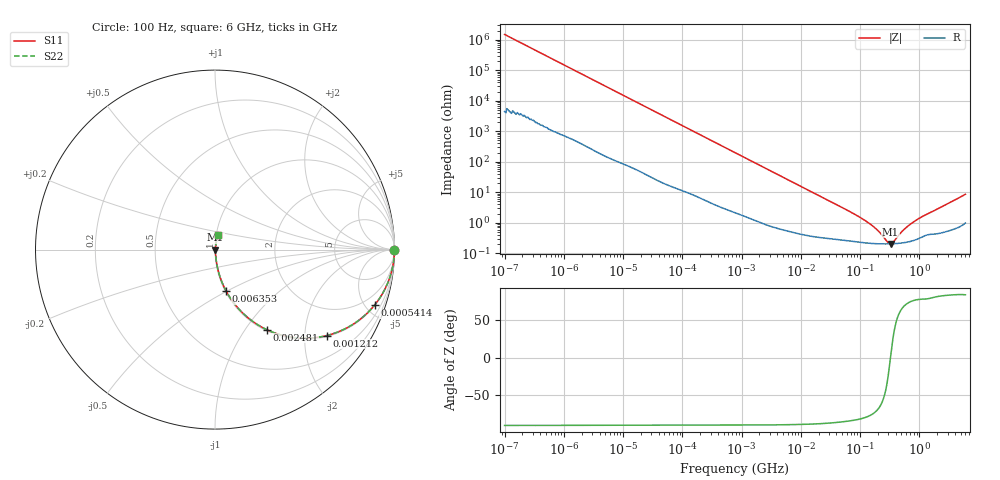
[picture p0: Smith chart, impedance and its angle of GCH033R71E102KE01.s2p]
!Murata Part Number: GCH033R71E102KE01
!These Parameters are Measured in Series Mode Connection
!Data Generated on Jun 19, 2026
!  o--ll--o
!Port1  Port2
!  o------o
!Operation Temp=25[degC], DC Bias Voltage=0[V]
!Freq. Start=100[Hz] Stop=6[GHz] 401[Steps]
# Hz S RI R 50
!Freq.(Hz) S11(Real) S11(Imag) S21(Real) S21(Imag) S12(Real) S12(Imag) S22(Real) S22(Imag)
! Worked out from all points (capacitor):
!   401 points, 100 Hz to 6 GHz, reference 50 ohm
!   read as one part in series: C = 1.06 nF near 109 Hz
!   lowest |Z| = 203 mohm at 326.7 MHz (marker M1)
!   series resonance near 326.3 MHz, so ESL is about 220 pH
!   S11 on the Smith chart (normalised r, x): 100 Hz: open; 541.4 kHz: 1.06, -5.73; 1.212 MHz: 1.03, -2.57; 2.481 MHz: 1.02, -1.26; 6.353 MHz: 1.01, -0.50; 6 GHz: 1.02, +0.17
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100  1 -6.66e-05  2e-07 6.66e-05  2e-07 6.66e-05  1 -6.66e-05
164  1 -0.000109  5e-07 0.000109  5e-07 0.000109  1 -0.000109
2008  1 -0.00132  8.5e-06 0.00132  8.5e-06 0.00132  1 -0.00132
40335  0.9991 -0.0263  0.000852 0.0263  0.000852 0.0263  0.9991 -0.0263
176758  0.9861 -0.113  0.0139 0.113  0.0139 0.113  0.9861 -0.113
541393  0.889 -0.3094  0.111 0.3094  0.111 0.3094  0.889 -0.3094
774597  0.7984 -0.3959  0.2016 0.3959  0.2016 0.3959  0.7984 -0.3959
1212075  0.6217 -0.4791  0.3783 0.4791  0.3783 0.4791  0.6217 -0.4791
1734173  0.4487 -0.491  0.5513 0.491  0.5513 0.491  0.4487 -0.491
2481164  0.2875 -0.4457  0.7125 0.4457  0.7125 0.4457  0.2875 -0.4457
3882480  0.1446 -0.3436  0.8554 0.3436  0.8554 0.3436  0.1446 -0.3436
6353432  0.0622 -0.2313  0.9378 0.2313  0.9378 0.2313  0.0622 -0.2313
1.555665e7  0.0137 -0.1  0.9863 0.1  0.9863 0.1  0.0137 -0.1
6.233367e7  0.00318 -0.0249  0.9968 0.0249  0.9968 0.0249  0.00318 -0.0249
1.220122e8  0.00231 -0.0115  0.9977 0.0115  0.9977 0.0115  0.00231 -0.0115
1.909225e8  0.00208 -0.00568  0.9979 0.00568  0.9979 0.00568  0.00208 -0.00568
3.124326e8  0.00203 -0.000439  0.998 0.000439  0.998 0.000439  0.00203 -0.000439
3.267395e8  0.00203 1.44e-05  0.998 -1.44e-05  0.998 -1.44e-05  0.00203 1.44e-05
3.737127e8  0.00206 0.00138  0.9979 -0.00138  0.9979 -0.00138  0.00206 0.00138
5.847788e8  0.00229 0.00624  0.9977 -0.00624  0.9977 -0.00624  0.00229 0.00624
8.749838e8  0.0029 0.0116  0.9971 -0.0116  0.9971 -0.0116  0.0029 0.0116
6e9  0.0168 0.0832  0.9832 -0.0832  0.9832 -0.0832  0.0168 0.0832
